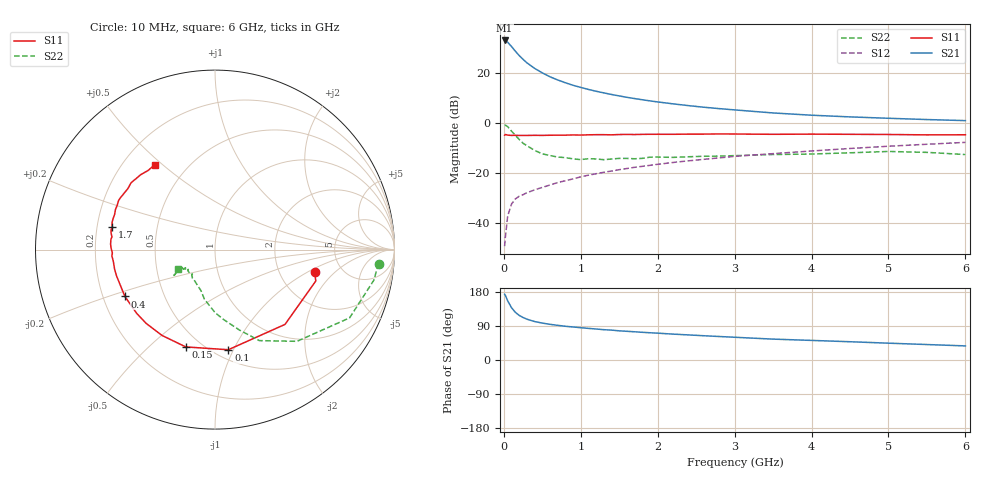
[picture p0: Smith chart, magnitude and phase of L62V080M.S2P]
!  INFINEON TECHNOLOGIES Small Signal Semiconductors
! BFR380L3 , Si-NPN RF-Transistor in TSLP-3-1
!  Vce=2 V,  Ic=80 mA
! Common Emitter S-Parameters:  07. March 2005
#  GHz  S  MA  R  50
! f  S11  S21  S12  S22
! GHz  Mag  Ang  Mag  Ang  Mag  Ang  Mag  Ang
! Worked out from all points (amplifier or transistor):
!   36 points, 10 MHz to 6 GHz, reference 50 ohm
!   highest |S21| = 32.8 dB at 10 MHz (marker M1)
!   |S21| within 3 dB of that: start of sweep to 115.4 MHz
!   unconditionally stable (mu >= 1): 1.103 GHz to 5.175 GHz
!   at 250 MHz: K = 0.56, MSG = 27.0 dB, |S12| = -28.6 dB
!   at 1.4 GHz: K = 1.04, MAG = 14.0 dB, |S12| = -19.2 dB
!   at 6 GHz: K = 0.98, MSG = 4.3 dB, |S12| = -7.8 dB
!   S11 on the Smith chart (normalised r, x): 10 MHz: 3.17, -1.16; 100 MHz: 0.59, -0.96; 150 MHz: 0.41, -0.66; 400 MHz: 0.29, -0.22; 1.7 GHz: 0.26, +0.10; 6 GHz: 0.33, +0.47
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0.01  0.5684 -12.6  43.9 173.5  0.0035 66.2  0.9143 -4.9
0.02  0.5882 -17.3  43.64 170.4  0.0053 73.2  0.9013 -10.9
0.05  0.5708 -46.9  40.51 156.1  0.014 71.1  0.8408 -26.9
0.1  0.5628 -82.4  33.22 138.0  0.0242 58.9  0.6855 -48.2
0.15  0.5662 -106.7  26.78 125.8  0.0306 53.5  0.5642 -64.0
0.2  0.562 -121.7  21.92 117.7  0.0347 52.0  0.4675 -73.2
0.25  0.5623 -133.0  18.45 112.1  0.0372 50.7  0.3924 -83.0
0.3  0.5626 -140.9  15.74 107.7  0.0407 51.6  0.352 -89.8
0.4  0.5658 -152.5  12.19 101.5  0.0463 52.9  0.2829 -102.0
0.5  0.5638 -160.0  9.923 97.4  0.0519 56.1  0.2421 -108.7
0.6  0.5677 -165.0  8.29 94.1  0.0579 58.0  0.2236 -115.4
0.7  0.57 -168.9  7.177 91.5  0.0648 60.3  0.2089 -122.2
0.9  0.5755 -176.5  5.61 87.1  0.0766 62.6  0.1921 -132.4
1.1  0.5789 179.2  4.642 83.4  0.0908 64.6  0.1937 -136.5
1.4  0.5783 173.0  3.683 78.9  0.11 66.0  0.1908 -142.0
1.7  0.5865 167.7  3.054 74.5  0.1303 66.5  0.193 -148.5
2.2  0.5926 160.7  2.395 68.3  0.1628 66.6  0.2056 -148.3
2.8  0.6029 152.9  1.925 62.0  0.201 66.3  0.2182 -152.4
3.5  0.5925 144.9  1.578 55.1  0.2441 64.0  0.2344 -150.2
4.5  0.5923 138.6  1.317 48.2  0.3093 61.8  0.2538 -148.8
5.5  0.5774 130.3  1.166 40.8  0.3753 57.7  0.2586 -148.7
6  0.5798 125.4  1.111 37.2  0.4092 55.4  0.2342 -152.1
